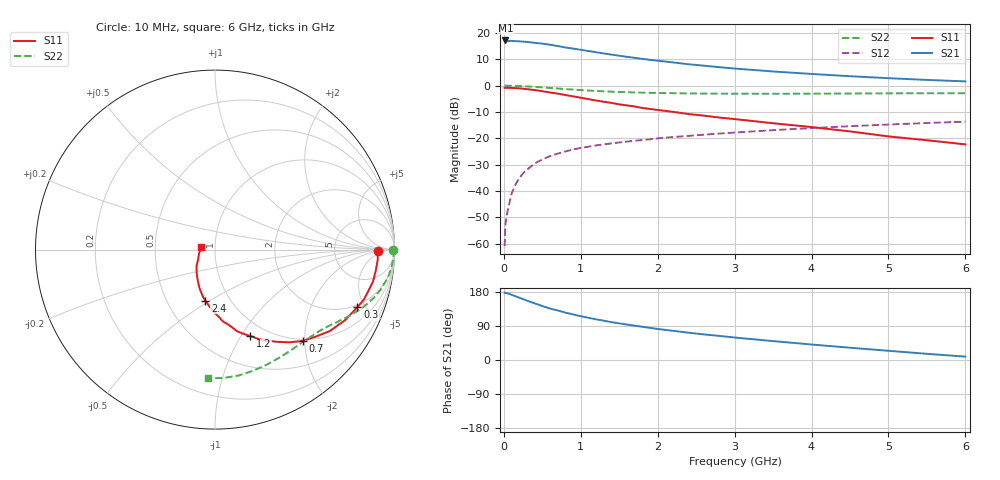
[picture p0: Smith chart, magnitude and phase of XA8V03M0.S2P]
! SIEMENS Discrete & RF Semiconductors
! BFY180
! Si NPN RF Bipolar Junction Transistor in MICRO-X
! VCE = 8 V  IC = 3 mA
! Common Emitter S-Parameters:  May  1997
# GHz  S  MA  R  50
!  f  S11  S21  S12  S22
! GHz  MAG  ANG  MAG  ANG  MAG  ANG  MAG  ANG
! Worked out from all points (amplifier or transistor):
!   36 points, 10 MHz to 6 GHz, reference 50 ohm
!   highest |S21| = 17.1 dB at 20 MHz (marker M1)
!   |S21| within 3 dB of that: start of sweep to 882.6 MHz
!   unconditionally stable (mu >= 1): 2.686 GHz to end of sweep
!   at 250 MHz: K = 0.16, MSG = 25.0 dB, |S12| = -33.3 dB
!   at 1.4 GHz: K = 0.73, MSG = 16.8 dB, |S12| = -21.9 dB
!   at 6 GHz: K = 1.06, MAG = 6.2 dB, |S12| = -13.7 dB
!   S11 on the Smith chart (normalised r, x): 10 MHz: 20, -2; 300 MHz: 1.84, -4.41; 700 MHz: 0.96, -1.95; 1.2 GHz: 0.83, -1.10; 2.4 GHz: 0.77, -0.48; 6 GHz: 0.86, +0.02
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0.01  0.9063 -0.6  7.172 177.7  0.0009 83.7  0.9935 -0.2
0.02  0.9064 -1.5  7.184 177.2  0.0023 86.8  0.9999 -0.7
0.05  0.9086 -3.5  7.016 175.8  0.0043 89.1  0.9955 -1.8
0.1  0.9031 -7.6  7.054 172.2  0.0089 87.0  0.9921 -3.7
0.2  0.8863 -14.7  6.917 164.4  0.0175 81.2  0.9826 -7.3
0.3  0.8559 -22.0  6.747 156.7  0.0253 76.8  0.9658 -10.8
0.5  0.7844 -35.3  6.258 142.4  0.0398 69.2  0.9254 -16.8
0.6  0.7412 -40.9  5.959 135.7  0.0459 66.2  0.9023 -19.4
0.7  0.7054 -46.2  5.625 130.8  0.0512 63.4  0.8811 -21.7
0.8  0.6633 -51.1  5.289 125.0  0.0563 61.0  0.8588 -23.8
1.1  0.5548 -64.0  4.523 111.4  0.0693 55.5  0.8056 -29.0
1.2  0.5208 -67.7  4.297 107.3  0.0734 53.9  0.7919 -30.6
1.4  0.4692 -75.1  3.872 99.9  0.0801 51.8  0.7673 -33.4
1.6  0.4208 -80.5  3.509 93.6  0.0867 50.2  0.7499 -36.0
2  0.3454 -91.3  2.971 81.9  0.0997 47.0  0.7252 -41.1
2.2  0.3177 -95.7  2.75 77.0  0.1058 45.3  0.7181 -43.7
2.4  0.289 -100.8  2.542 72.1  0.1111 44.1  0.7107 -46.1
3  0.2318 -111.9  2.106 59.3  0.1286 40.1  0.7025 -53.3
3.5  0.1932 -120.2  1.854 49.9  0.1428 36.8  0.7007 -59.5
4.5  0.1353 -139.3  1.507 32.4  0.1697 29.8  0.7075 -72.3
5.5  0.0919 -166.1  1.282 16.3  0.1953 22.0  0.7169 -86.1
6  0.0768 170.4  1.202 8.9  0.2068 17.9  0.7177 -93.1
